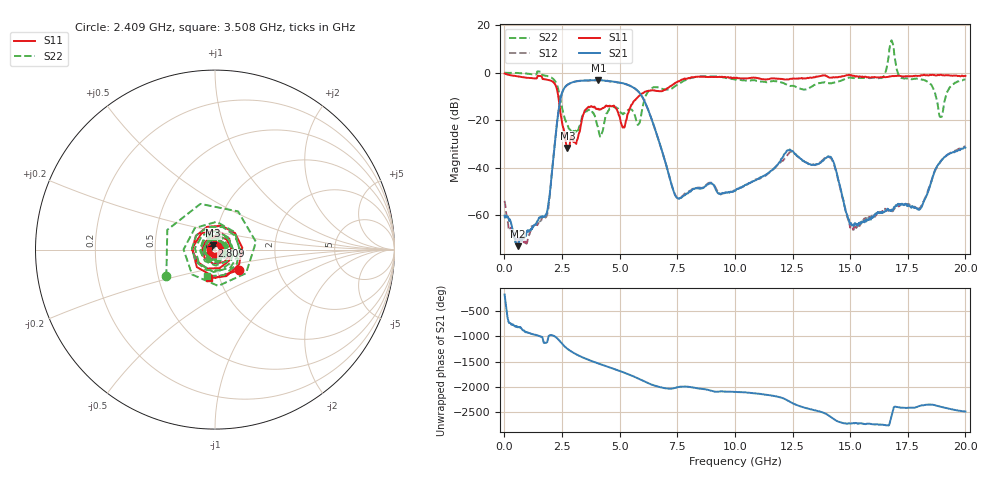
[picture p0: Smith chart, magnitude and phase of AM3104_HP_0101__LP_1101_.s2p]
!Created with skrf (http://scikit-rf.org).
# Hz S RI R 50.0
!freq ReS11 ImS11 ReS21 ImS21 ReS12 ImS12 ReS22 ImS22
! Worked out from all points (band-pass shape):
!   1601 points, 10 MHz to 20 GHz, reference 50 ohm
!   highest |S21| = -3.15 dB at 4.083 GHz (marker M1); lowest = -73.1 dB at 584.7 MHz (marker M2)
!   |S21| within 3 dB of the highest: 2.624 GHz to 5.582 GHz (2.958 GHz wide, 72.1 % of centre)
!   lowest |S11| = -31.7 dB at 2.734 GHz (marker M3), VSWR 1.05, Z = 49 + j2.36 ohm
!   |S11| at or under -10 dB: 2.339 GHz to 5.817 GHz (3.477 GHz wide, 85.3 % of centre)
!   |S22| runs from -27.1 to 13.6 dB; largest |S21 - S12| = 0.07
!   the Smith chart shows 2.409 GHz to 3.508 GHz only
!   S11 on the Smith chart (normalised r, x): 2.409 GHz: 1.27, -0.30; 2.809 GHz: 0.96, +0.04; 3.508 GHz: 0.89, -0.29
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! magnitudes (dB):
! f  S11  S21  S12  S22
! 10 MHz  -0.4  -60.3  -54.0  0.0
! 584.7 MHz  -1.6  -73.1  -70.4  -0.1
! 1.834 GHz  -2.9  -59.2  -60.3  -1.3
! 2.409 GHz  -15.1  -12.3  -12.4  -10.2
! 2.734 GHz  -31.7  -5.1  -5.1  -22.1
! 2.809 GHz  -31.6  -4.6  -4.7  -23.7
! 3.346 GHz  -20.6  -3.4  -3.4  -19.7
! 3.508 GHz  -15.8  -3.3  -3.3  -16.2
! 4.083 GHz  -15.2  -3.2  -3.2  -24.3
! 5.157 GHz  -22.9  -4.5  -4.5  -17.4
! 5.782 GHz  -10.4  -7.6  -7.7  -21.9
! 6.682 GHz  -7.7  -28.0  -28.1  -6.2
! 7.506 GHz  -3.9  -52.8  -52.9  -5.1
! 10.01 GHz  -2.3  -49.8  -49.7  -2.9
! 12.33 GHz  -2.8  -32.7  -34.2  -5.5
! 13.34 GHz  -2.2  -38.9  -38.8  -5.8
! 14.2 GHz  -2.1  -36.2  -36.6  -4.4
! 15.06 GHz  -1.1  -64.2  -65.2  -2.1
! 16.68 GHz  -1.6  -57.9  -58.3  7.3
! 18.04 GHz  -1.4  -57.5  -57.0  -2.8
! 18.93 GHz  -0.8  -37.3  -37.4  -18.6
! 20 GHz  -1.3  -31.6  -31.0  -2.8
